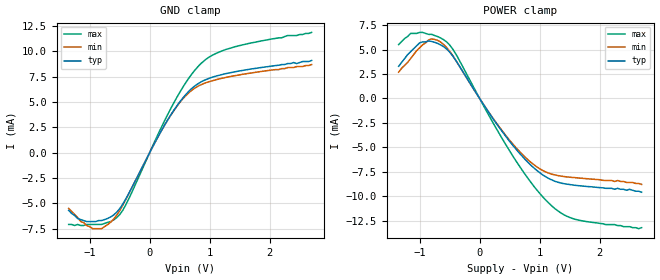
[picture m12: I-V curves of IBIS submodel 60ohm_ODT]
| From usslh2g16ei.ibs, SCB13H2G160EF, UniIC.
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| SUBMODEL 60ohm_ODT
[Submodel]   60ohm_ODT
Submodel_type  Dynamic_clamp
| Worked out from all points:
|   GND clamp passes 1 mA (typ) near -0.09 V on its own axis
|   POWER clamp passes 1 mA (typ) near -0.10 V on its own axis
[GND Clamp]
|Voltage   I(typ)   I(min)   I(max)
-1.35V    -5.7mA     -5.5mA     -7.083mA
-1.2V     -6.5mA     -6.4mA     -7.083mA
-950mV    -6.8mA     -7.5mA     -7.083mA
-800mV    -6.7mA     -7.5mA     -7.083mA
-650mV    -6.34mA    -6.86mA    -6.802mA
-400mV    -4.59mA    -4.65mA    -5.177mA
100mV     1.138mA    1.137mA    1.308mA
400mV     4.16mA     4.12mA     4.885mA
650mV     6.04mA     5.9mA      7.333mA
950mV     7.24mA     6.93mA     9.271mA
1.45V     8.02mA     7.63mA     10.5mA
2.7V      9.1mA      8.7mA      11.88mA
[POWER Clamp]
|Voltage   I(typ)   I(min)   I(max)
-1.35V    3.3mA      2.7mA      5.521mA
-1.15V    4.8mA      4.1mA      6.667mA
-1V       5.7mA      5.2mA      6.771mA
-850mV    5.9mA      6mA        6.562mA
-700mV    5.64mA     5.95mA     6.344mA
-550mV    5.07mA     5.22mA     5.792mA
-400mV    3.92mA     3.93mA     4.594mA
500mV     -4.4mA     -4.28mA    -5.365mA
850mV     -6.81mA    -6.52mA    -8.552mA
1.2V      -8.33mA    -7.75mA    -10.99mA
1.6V      -8.9mA     -8.11mA    -12.39mA
2.7V      -9.6mA     -8.8mA     -13.23mA
